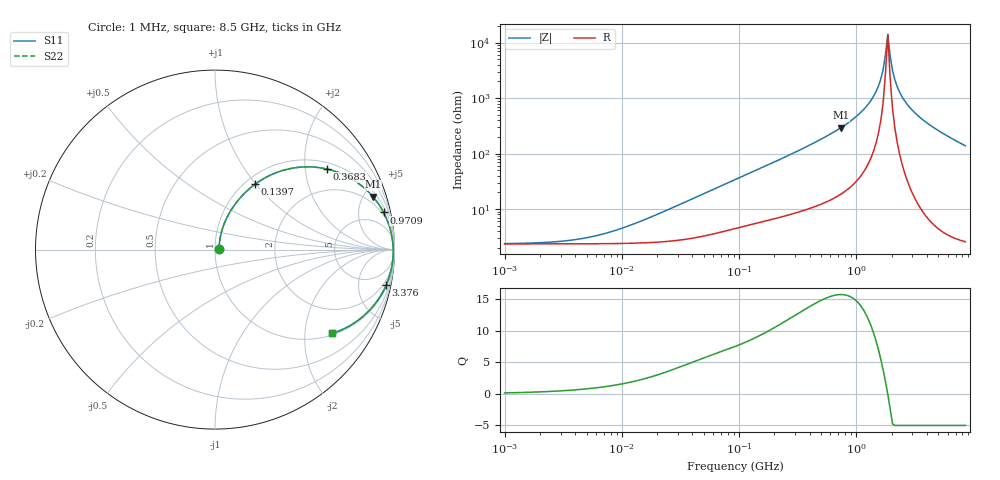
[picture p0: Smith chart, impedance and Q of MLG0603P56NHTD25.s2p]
! S-Parameter Data Generated by TDK Corporation
! Copyright(C) 2025 TDK Corporation.
! All Rights Reserved.
! TDK P/N: MLG0603P56NHTD25 (SMD / SMT Inductor (Coil))
! Property: L=56nH at 300MHz
! Size(LxWxT): 0.6x0.3x0.3mm
! Model Type: s2p (Touchstone File Format Version 1.0)
! Frequency: DC=Yes Start=1MHz Stop=8500MHz 198points Log-sweep
! Model Generated on Feb. 6, 2025
! Terms and conditions regarding TDK Simulation Models:
! 1)This simulation model is being provided solely for informational
!  purposes. Please refer to the specifications of the products in
!  terms of detailed characteristics of such products.
! 2)In no event shall TDK Corporation of any of its subsidiaries be
!  liable for any loss or damage arising, directly or indirectly,
!  from any information contained in this simulation model, including,
!  but not limited to loss or damages arising from any inaccuracies,
!  omissions or errors in connection with such information.
! 3)Any and all copyrights on this simulation model are owned by
!  TDK Corporation.  Duplication or redistribution of this simulation
!  model without prior written permission from TDK Corporation
!  is prohibited.
! 4)This simulation model is subject to any modification or change
!  without any prior notice.
! 5)Neither TDK Corporation nor any of its subsidiaries shall make any
!  warranty, express or implied, including but not limited to the
!  correctness, implied warranties of merchantability and fitness for
!  a particular purpose with respect to this simulation models.
! 6)The use of this simulation model shall be deemed to have consented
!  to the terms and conditions hereof.
! Port Assignments:
!  1 ---@@@--- 2
! Applicable Conditions:
!  Temperature = 25 degC
!  DC Bias Current = 0 A
!  Small Signal Operation
# Hz S MA R 50
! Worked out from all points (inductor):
!   197 points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, 1 MHz to 8.5 GHz, reference 50 ohm
!   read as one part in series: L = 60.4 nH near 20.1 MHz
!   highest Q = 15.8 at 736 MHz (marker M1), where L = 63.1 nH
!   self-resonance near 1.769 GHz
!   S11 on the Smith chart (normalised r, x): 1 MHz: 1.05, +0.01; 139.7 MHz: 1.11, +0.99; 368.3 MHz: 1.19, +2.61; 970.9 MHz: 1.59, +8.90; 3.376 GHz: 1.24, -9.50; 8.5 GHz: 1.05, -2.77
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1000000  0.02327 9.0  0.977 -0.2  0.977 -0.2  0.02327 9.0
4587603  0.02871 35.6  0.9768 -1.0  0.9768 -1.0  0.02871 35.6
9168677  0.04136 53.7  0.9761 -2.0  0.9761 -2.0  0.04136 53.7
2.10461e7  0.08163 67.9  0.9722 -4.5  0.9722 -4.5  0.08163 67.9
9.219544e7  0.3078 64.7  0.9118 -17.8  0.9118 -17.8  0.3078 64.7
1.396825e8  0.4289 58.4  0.8571 -25.2  0.8571 -25.2  0.4289 58.4
3.682571e8  0.7676 35.8  0.5867 -49.9  0.5867 -49.9  0.7676 35.8
4.229561e8  0.8089 32.2  0.5337 -53.8  0.5337 -53.8  0.8089 32.2
7.359901e8  0.9285 18.5  0.3173 -67.9  0.3173 -67.9  0.9285 18.5
9.708683e8  0.9622 12.4  0.2159 -73.7  0.2159 -73.7  0.9622 12.4
1.280704e9  0.9824 6.9  0.1207 -78.2  0.1207 -78.2  0.9824 6.9
1.540426e9  0.9898 3.4  0.06001 -78.5  0.06001 -78.5  0.9898 3.4
1.689417e9  0.9919 1.7  0.03034 -73.7  0.03034 -73.7  0.9919 1.7
1.852819e9  0.993 -0.0  0.007043 5.3  0.007043 5.3  0.993 -0.0
1.940355e9  0.9932 -0.9  0.01707 65.9  0.01707 65.9  0.9932 -0.9
2.032026e9  0.9931 -1.8  0.03143 76.4  0.03143 76.4  0.9931 -1.8
2.128028e9  0.9927 -2.6  0.04632 79.6  0.04632 79.6  0.9927 -2.6
2.333852e9  0.9912 -4.4  0.07666 81.3  0.07666 81.3  0.9912 -4.4
2.680511e9  0.987 -7.1  0.1233 80.4  0.1233 80.4  0.987 -7.1
3.37643e9  0.9737 -11.8  0.2048 76.7  0.2048 76.7  0.9737 -11.8
5.115526e9  0.9243 -21.5  0.3664 67.5  0.3664 67.5  0.9243 -21.5
8.5e9  0.8035 -35.5  0.5805 53.5  0.5805 53.5  0.8035 -35.5
